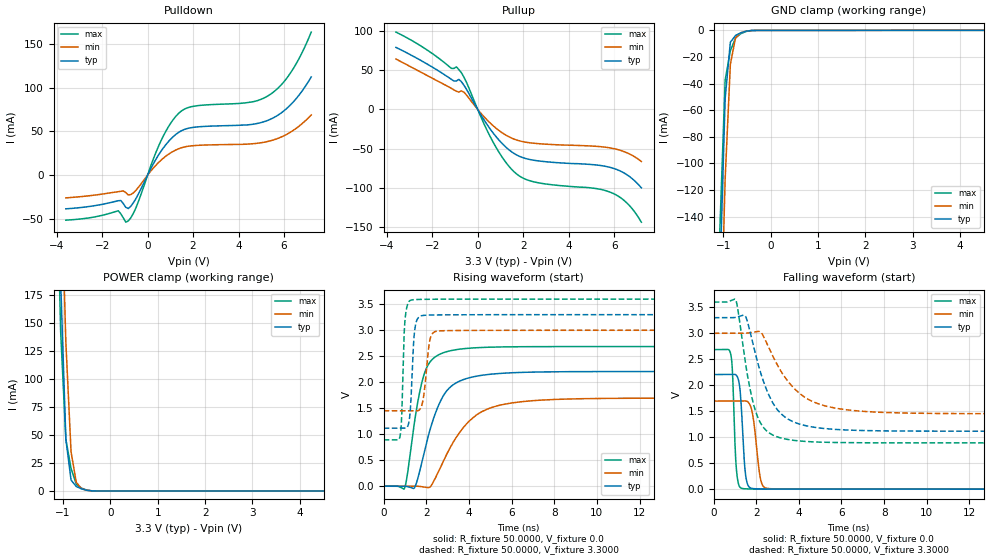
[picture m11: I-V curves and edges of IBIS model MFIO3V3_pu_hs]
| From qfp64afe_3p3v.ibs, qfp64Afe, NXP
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[Model] MFIO3V3_pu_hs
|   Model MFIO3V3_pu_hs
| This model was characterised for following simulation conditions:
| External (pad) voltage:
|   - Typ: 3.3V,   - Min: 3.0V,   - Max: 3.6V
| Library cells for typ/min/max conditions are connected as defined below:
|  IO - External Pad
|  A - Core Input
|  EN - Output Buffer Enable
|  BOOST - vdde
|  EHS - vdd
|  ENZI - vdd
|  EPD - gnd
|  EPUN - gnd
|  ZI - NC
|  ZIF - NC
|  gnd - gnd
|  gnde - gnde
|  vdd - vdd
|  vdde - vdde
| All other pins connected to ground
Model_type I/O
Polarity   Non-Inverting
Enable   Active-Low
Vinl =   0.9900V
Vinh =   2.3100V
Vmeas =  1.6500V
Cref =   0.0F
Rref =   100.0000
Vref =   0.0V
C_comp   1.5343pF   1.4580pF   1.6019pF
|C_comp_pullup   0.7259pF   0.7507pF   0.6892pF
|C_comp_pulldown   0.5955pF   0.6341pF   0.5597pF
[Model Spec]
| variable   typ   min   max
Vinh   0.9900V   0.9000V   1.0800V
Vinl   2.3100V   2.1000V   2.5200V
Vmeas   1.6500V   1.5000V   1.8000V
[Temperature Range]   25.0000   0.1250k   -40.0000
[Voltage Range]   3.3000V   3.0000V   3.6000V
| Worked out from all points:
|   slope of the pulldown table from 0 to 0.495 V, typ, clamps not added: 21 ohm
|   slope of the pullup table from 0 to 0.495 V, typ, clamps not added: 21.7 ohm
|   GND clamp passes 1 mA (typ) near -0.55 V on its own axis
|   POWER clamp passes 1 mA (typ) near -0.54 V on its own axis
|   rising waveform, R_fixture 50.0000, V_fixture 0.0: 20-80 % time 1.06ns typ, 1.67ns min, 677ps max; typ from 0.001 V to 2.21 V
|   rising waveform, R_fixture 50.0000, V_fixture 3.3000: 20-80 % time 158ps typ, 234ps min, 124ps max; typ from 1.12 V to 3.3 V
|   falling waveform, R_fixture 50.0000, V_fixture 0.0: 20-80 % time 188ps typ, 278ps min, 145ps max; typ from 2.21 V to 0.001 V
|   falling waveform, R_fixture 50.0000, V_fixture 3.3000: 20-80 % time 1.14ns typ, 1.68ns min, 749ps max; typ from 3.3 V to 1.12 V
[Pulldown]
|Voltage   I(typ)   I(min)   I(max)
-3.6V     -38.54mA   -26.03mA   -51.47mA
-1.29V    -29.27mA   -18.96mA   -40.78mA
-960mV    -36.81mA   -20.01mA   -53.83mA
-850mV    -38.18mA   -22.68mA   -52.4mA
-520mV    -27.12mA   -17.5mA    -37.74mA
580mV     26.98mA    16.83mA    38.78mA
1.35V     48.62mA    30.01mA    70.27mA
2.01V     54.62mA    33.69mA    78.71mA
4.43V     57.57mA    35.54mA    83.11mA
5.31V     62.85mA    38.64mA    90.87mA
6.3V      80.67mA    49.35mA    117.4mA
7.2V      112.3mA    68.85mA    163.6mA
[Pullup]
|Voltage   I(typ)   I(min)   I(max)
-3.6V     79.43mA    64.59mA    99.03mA
-1.05V    36.46mA    25.05mA    52.51mA
-830mV    38.41mA    22.29mA    50.98mA
-610mV    31.13mA    22.16mA    41.54mA
270mV     -13.03mA   -9.075mA   -18mA
710mV     -31.29mA   -21.6mA    -43.53mA
1.26V     -48.73mA   -33.16mA   -68.54mA
1.7V      -58.01mA   -38.97mA   -82.27mA
2.58V     -65.44mA   -43.49mA   -93.28mA
5.88V     -74.5mA    -49.46mA   -106.4mA
6.65V     -85.18mA   -56.54mA   -122.1mA
7.2V      -100.2mA   -66.51mA   -144.2mA
[GND_clamp]
|Voltage   I(typ)   I(min)   I(max)
-3.6V     -4.776A    -4.755A    -4.803A
-1.07V    -185.3mA   -255.8mA   -148mA
-960mV    -51.33mA   -111.9mA   -37.44mA
-850mV    -8.945mA   -25.5mA    -15.28mA
-740mV    -3.847mA   -5.583mA   -5.729mA
-630mV    -1.869mA   -1.835mA   -2.528mA
-520mV    -657.8uA   -634.6uA   -865.1uA
-300mV    -74.33uA   -64.35uA   -93.3uA
7.2V      0A         0A         0A
[POWER_clamp]
|Voltage   I(typ)   I(min)   I(max)
-3.6V     5.691A     5.665A     5.731A
-1.16V    387.4mA    485.6mA    339.2mA
-1.05V    187.8mA    295.9mA    142.7mA
-940mV    46.36mA    133mA      46.18mA
-830mV    9.713mA    34.98mA    20.13mA
-720mV    3.977mA    7.725mA    5.963mA
-610mV    1.851mA    2.026mA    2.529mA
-500mV    580.4uA    628.9uA    748uA
-280mV    7.181uA    13.64uA    7.137uA
7.2V      0A         0A         0A
[Ramp]
| variable   typ   min   max
dV/dt_r  1.3233/1.0567n   1.0168/1.6724n   1.6114/0.6769n
dV/dt_f  1.3106/1.1404n   0.9289/1.6819n   1.6253/0.7486n
R_load = 50.0000
[Rising Waveform]
R_fixture= 50.0000
V_fixture= 0.0
V_fixture_min= 0.0
V_fixture_max= 0.0
|time   V(typ)   V(min)   V(max)
0s        878.6uV    956.8uV    853.3uV
985.3ps   944.4uV    930.3uV    -31.89mV
1.464ns   -17.36mV   1.213mV    1.282V
1.785ns   451.8mV    -8.819mV   1.987V
2.13ns    1.022V     -24.79mV   2.364V
2.955ns   1.833V     613mV      2.588V
4.216ns   2.106V     1.327V     2.661V
6.045ns   2.183V     1.604V     2.682V
10.54ns   2.206V     1.69V      2.686V
100ns     2.206V     1.696V     2.686V
[Rising Waveform]
R_fixture= 50.0000
V_fixture= 3.3000
V_fixture_min= 3.0000
V_fixture_max= 3.6000
|time   V(typ)   V(min)   V(max)
0s        1.116V     1.452V     891.1mV
782.1ps   1.116V     1.452V     989.1mV
847.9ps   1.116V     1.452V     1.369V
976.5ps   1.114V     1.452V     3.05V
1.151ns   1.176V     1.452V     3.527V
1.456ns   3.002V     1.45V      3.59V
1.834ns   3.284V     1.633V     3.595V
2.216ns   3.293V     2.882V     3.597V
2.761ns   3.296V     2.99V      3.598V
100ns     3.3V       3V         3.6V
[Falling Waveform]
R_fixture= 50.0000
V_fixture= 0.0
V_fixture_min= 0.0
V_fixture_max= 0.0
|time   V(typ)   V(min)   V(max)
0s        2.206V     1.696V     2.686V
802.3ps   2.206V     1.696V     2.588V
882.1ps   2.207V     1.696V     2.226V
1.076ns   2.185V     1.696V     323.9mV
1.241ns   1.882V     1.696V     33.36mV
1.446ns   474mV      1.699V     8.466mV
1.8ns     15.13mV    1.495V     4.074mV
2.241ns   4.975mV    125.3mV    2.663mV
2.705ns   3.174mV    8.723mV    1.968mV
100ns     878.6uV    956.8uV    853.3uV
[Falling Waveform]
R_fixture= 50.0000
V_fixture= 3.3000
V_fixture_min= 3.0000
V_fixture_max= 3.6000
|time   V(typ)   V(min)   V(max)
0s        3.3V       3V         3.6V
1.046ns   3.308V     3V         3.631V
1.508ns   3.314V     3.002V     2.378V
1.851ns   2.782V     3.02V      1.66V
2.245ns   2.183V     3.004V     1.24V
3.04ns    1.504V     2.352V     999mV
4.32ns    1.222V     1.758V     918.9mV
6.342ns   1.138V     1.523V     895.5mV
10.35ns   1.117V     1.458V     891.2mV
100ns     1.116V     1.452V     891.1mV
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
